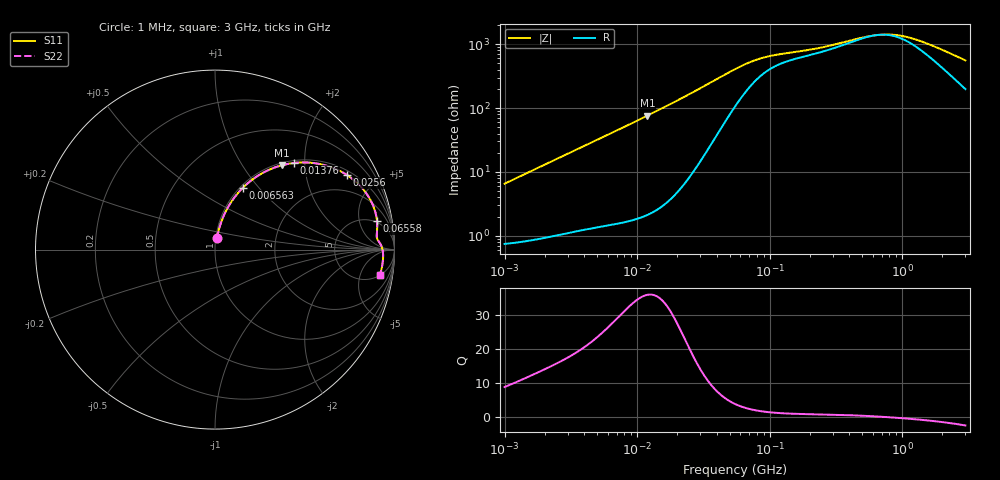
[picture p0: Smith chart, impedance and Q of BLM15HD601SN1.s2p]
! BLM15HD601SN1
# Hz S RI R 50
!Freq.(Hz) S11(Real) S11(Imag) S21(Real) S21(Imag) S12(Real) S12(Imag) S22(Real) S22(Imag)
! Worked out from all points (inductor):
!   401 points, 1 MHz to 3 GHz, reference 50 ohm
!   read as one part in series: L = 1.03 uH near 1.041 MHz
!   highest Q = 36 at 11.96 MHz (marker M1), where L = 1.01 uH
!   self-resonance near 655.7 MHz
!   S11 on the Smith chart (normalised r, x): 1 MHz: 1.01, +0.13; 6.563 MHz: 1.03, +0.83; 13.76 MHz: 1.05, +1.76; 25.6 MHz: 1.18, +3.42; 65.58 MHz: 5, +9; 3 GHz: 5, -10
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1000000  0.0115 0.0638  0.9885 -0.0638  0.9885 -0.0638  0.0115 0.0638
2055611  0.0261 0.1279  0.9739 -0.1279  0.9739 -0.1279  0.0261 0.1279
3823119  0.0661 0.2247  0.9339 -0.2247  0.9339 -0.2247  0.0661 0.2247
6563319  0.1563 0.3456  0.8437 -0.3456  0.8437 -0.3456  0.1563 0.3456
8861669  0.2467 0.4161  0.7533 -0.4161  0.7533 -0.4161  0.2467 0.4161
1.196486e7  0.3714 0.4695  0.6286 -0.4695  0.6286 -0.4695  0.3714 0.4695
1.37644e7  0.4391 0.4825  0.5609 -0.4825  0.5609 -0.4825  0.4391 0.4825
1.461624e7  0.4692 0.485  0.5308 -0.485  0.5308 -0.485  0.4692 0.485
1.896016e7  0.6008 0.473  0.3992 -0.473  0.3992 -0.473  0.6008 0.473
2.559965e7  0.7354 0.4155  0.2646 -0.4155  0.2646 -0.4155  0.7354 0.4155
3.670325e7  0.8444 0.3114  0.1556 -0.3114  0.1556 -0.3114  0.8444 0.3114
5.477226e7  0.8957 0.1995  0.1043 -0.1995  0.1043 -0.1995  0.8957 0.1995
6.558369e7  0.9024 0.1601  0.0976 -0.1601  0.0976 -0.1601  0.9024 0.1601
8.173662e7  0.9038 0.1232  0.0962 -0.1232  0.0962 -0.1232  0.9038 0.1232
9.984923e7  0.9024 0.0991  0.0976 -0.0991  0.0976 -0.0991  0.9024 0.0991
2.094008e8  0.9062 0.0551  0.0938 -0.0551  0.0938 -0.0551  0.9062 0.0551
5.473095e8  0.9305 0.0107  0.0695 -0.0107  0.0695 -0.0107  0.9305 0.0107
6.685918e8  0.9336 -0.0012  0.0664 0.0012  0.0664 0.0012  0.9336 -0.0012
8.005644e8  0.9355 -0.0128  0.0645 0.0128  0.0645 0.0128  0.9355 -0.0128
1.017911e9  0.9367 -0.0296  0.0633 0.0296  0.0633 0.0296  0.9367 -0.0296
1.320433e9  0.9363 -0.0502  0.0637 0.0502  0.0637 0.0502  0.9363 -0.0502
3e9  0.9177 -0.1442  0.0823 0.1442  0.0823 0.1442  0.9177 -0.1442
